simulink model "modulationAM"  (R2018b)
settings: Solver=ode4  StartTime=0.0  StopTime=0.1  FixedStep=Ts  RelTol=1e-3  EnableMultiTasking=on
InitFcn:
  | omega0=500;
  | m=1;
  | Ts=1e-4;
libraries: simulink_extras x3, commchan3 x1

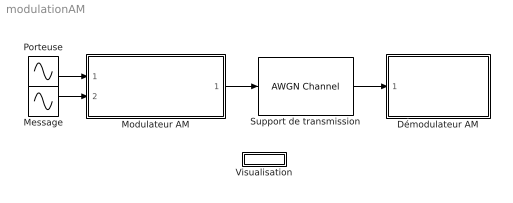
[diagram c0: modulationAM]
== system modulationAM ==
  Démodulateur AM : Subsystem
  Message : Sin  Amplitude=2  Frequency=500
  Modulateur AM : Subsystem
  Porteuse : Sin  Frequency=5000  SampleTime=0
  Support de transmission : commchan3/AWGN Channel  InputProcessing=Columns as channels (frame based)  seed=67  noiseMode="Signal to noise ratio  (SNR)"  EbNodB=15  EsNodB=10  SNRdB=60  bitsPerSym=4  Ps=1  Tsym=0.001  variance=1
  Visualisation : Subsystem
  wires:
  Porteuse/1 -> Modulateur AM/1(Porteuse)
  Message/1 -> Modulateur AM/2(Message)
  Modulateur AM/1(Signal modulé AM) -> Support de transmission/1
  Support de transmission/1 -> Démodulateur AM/1(Signal modulé reçu)

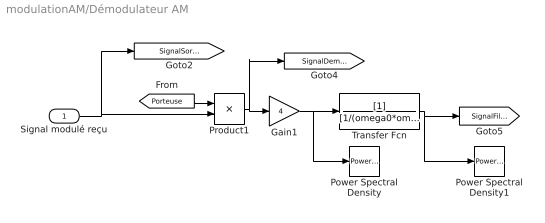
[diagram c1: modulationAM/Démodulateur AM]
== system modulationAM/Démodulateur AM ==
  Signal modulé reçu : Inport
  Gain1 : Gain  Gain=4
  Power Spectral Density : simulink_extras/Additional Sinks/Power Spectral Density  npts=2048  fftpts=2048  HowOften=1024  sampleT=Ts
  Power Spectral Density1 : simulink_extras/Additional Sinks/Power Spectral Density  npts=2048  fftpts=2048  HowOften=1024  sampleT=Ts
  Product1 : Product
  Transfer Fcn : TransferFcn  Denominator=[1/(omega0*omega0) 2*m/omega0 1]
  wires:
  Product1/1 -> [SignalDemodule], Gain1/1
  Transfer Fcn/1 -> Power Spectral Density1/1, [SignalFiltre]
  Signal modulé reçu/1 -> [SignalSortieCanal], Product1/2
  Gain1/1 -> Power Spectral Density/1, Transfer Fcn/1
  [Porteuse] -> Product1/1

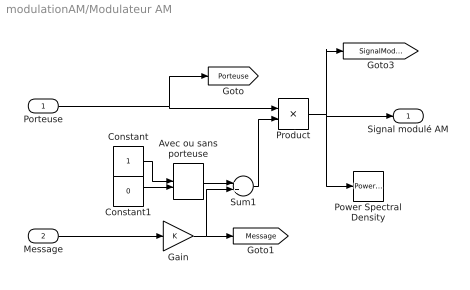
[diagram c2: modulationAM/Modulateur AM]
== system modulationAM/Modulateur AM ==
  Porteuse : Inport
  Message : Inport  Port=2
  Avec ou sans porteuse : ManualSwitch
  Constant : Constant
  Constant1 : Constant  Value=0
  Gain : Gain
  Power Spectral Density : simulink_extras/Additional Sinks/Power Spectral Density  npts=2048  fftpts=2048  HowOften=1024  sampleT=Ts
  Product : Product
  Sum1 : Sum
  Signal modulé AM : Outport
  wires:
  Constant/1 -> Avec ou sans porteuse/1
  Porteuse/1 -> [Porteuse], Product/1
  Product/1 -> Signal modulé AM/1, [SignalModule], Power Spectral Density/1
  Avec ou sans porteuse/1 -> Sum1/1
  Sum1/1 -> Product/2
  Message/1 -> Gain/1
  Gain/1 -> [Message], Sum1/2
  Constant1/1 -> Avec ou sans porteuse/2

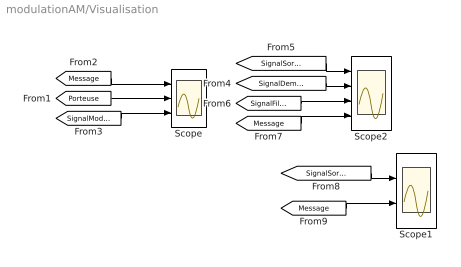
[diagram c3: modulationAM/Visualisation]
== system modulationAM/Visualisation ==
  Scope : Scope  NumInputPorts=3
  Scope1 : Scope  NumInputPorts=2
  Scope2 : Scope  NumInputPorts=4
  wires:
  [Message] -> Scope/1
  [SignalSortieCanal] -> Scope2/1
  [Porteuse] -> Scope/2
  [SignalModule] -> Scope/3
  [SignalDemodule] -> Scope2/2
  [SignalFiltre] -> Scope2/3
  [Message] -> Scope2/4
  [SignalSortieCanal] -> Scope1/1
  [Message] -> Scope1/2
